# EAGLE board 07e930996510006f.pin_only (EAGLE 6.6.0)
REV: B

Size 45 x 85 mm. Coordinates in mm from the lower left corner, seen from the top.
Outline: 0,3 0,82 arc-90 3,85 42,85 arc-90 45,82 45,3 arc-90 42,0 3,0 arc-90 0,3
Copper layers (1*16): Top 0.035mm / dielectric 1.5mm / Bottom 0.035mm
Design rules "adafruit": minimum track width 8mil, minimum drill 15.5mil, track to track 8mil, track to pad 8mil, pad to pad 8mil, via to via 8mil, smd to smd 8mil, copper to edge 10mil, drill to drill 8mil, minimum pad ring 10mil, minimum via ring 8mil, stop-mask expansion 4mil, vias tented up to drill 20mil, thermal gap 10mil
tRestrict: area 31.5,16.2 to 31.9,16.3; area 4.2,24.6 to 4.5,24.6; area 4.2,31.8 to 4.6,31.9; area 4.2,16.8 to 4.6,16.9; area 4.2,16.2 to 4.6,16.2

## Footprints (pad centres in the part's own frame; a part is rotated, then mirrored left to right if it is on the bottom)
_0805 = smd 1.2 x 1.3: 1 -1.016,0; 2 1.016,0
PANASONIC_C = smd 2.6 x 1.4: + 2.05,0; - -2.05,0
POWERDI-5 = smd 1.39 x 1.4: A1 -0.92,-2.84; A2 0.92,-2.84 | smd 3.36 x 4.86: C 0,1.142
SOD-323 = smd 1.35 x 0.8: A 1.27,0; C -1.27,0
FIDUCIAL_1MM = smd 1 x 1: 1 0,0
SOIC8 = smd 0.5 x 2.2: 1 -1.905,-3.154; 2 -0.645,-3.154; 3 0.625,-3.154; 4 1.895,-3.154; 5 1.905,3.154; 6 0.635,3.154; 7 -0.635,3.154; 8 -1.905,3.154
AVRISP = drill 0.9 pad 1.626: 1 -1.27,2.54; 2 1.27,2.54; 3 -1.27,0; 4 1.27,0; 5 -1.27,-2.54; 6 1.27,-2.54
1X01-CLEANBIG = drill 1.016 pad 1.778: 1 0,0
INDUCTOR_6X6MM_SUMIDA_CDRH5D28 = smd 3 x 6.5: P$1 -2.075,0; P$2 2.075,0
INDUCTOR_5X5MM_TDK_VLC5045 = smd 2.54 x 5: P$1 -2.096,0; P$2 2.096,0
CHIPLED_0805 = smd 1.2 x 1.2: A 0,-1.05; C 0,1.05
EG1390 = smd 1 x 1.5: O1 -2.5,2.8; O2 -2.5,-2.8; P1 0,2.8; P2 0,-2.8; S1 2.5,2.8; S2 2.5,-2.8 | hole 1: 1.5,0; -1.5,0
DPAK = smd 1.6 x 2.997: 1 -2.261,-4.928; 3 2.21,-4.928 | smd 5.452 x 7: 4 0,1.853
_0805MP = smd 1.2 x 1.3: 1 -1.016,0; 2 1.016,0
2512 = smd 1.8 x 3.2: 1 -2.8,0; 2 2.8,0
SOLDERJUMPER_2WAY_OPEN_NOPASTE = smd 1.168 x 1.6: 1 -1.397,0; 2 0,0; 3 1.397,0
EVQ-Q2 = smd 3.2 x 1.2: A -3.4,-2; A' 3.4,-2; B -3.4,2; B' 3.4,2
SOT-23 = smd 0.787 x 0.889: 1 0.025,-1.016; 2 -0.94,1.016; 3 0.991,1.016
TESTPOINT_ROUND_1MM = smd 1 x 1: P$1 0,0
QFN32_5MM = smd 0.8 x 0.25: 1 -2.5,1.75; 2 -2.5,1.25; 3 -2.5,0.75; 4 -2.5,0.25; 5 -2.5,-0.25; 6 -2.5,-0.75; 7 -2.5,-1.25; 8 -2.5,-1.75; 17 2.5,-1.75; 18 2.5,-1.25; 19 2.5,-0.75; 20 2.5,-0.25; 21 2.5,0.25; 22 2.5,0.75; 23 2.5,1.25; 24 2.5,1.75 | smd 0.25 x 0.8: 9 -1.75,-2.5; 10 -1.25,-2.5; 11 -0.75,-2.5; 12 -0.25,-2.5; 13 0.25,-2.5; 14 0.75,-2.5; 15 1.25,-2.5; 16 1.75,-2.5; 25 1.75,2.5; 26 1.25,2.5; 27 0.75,2.5; 28 0.25,2.5; 29 -0.25,2.5; 30 -0.75,2.5; 31 -1.25,2.5; 32 -1.75,2.5 | smd 3.5 x 3.5: 33 0,0
QFN16_3MM = smd 0.8 x 0.28: 1 -1.5,0.75; 2 -1.5,0.25; 3 -1.5,-0.25; 4 -1.5,-0.75; 9 1.5,-0.75; 10 1.5,-0.25; 11 1.5,0.25; 12 1.5,0.75 | smd 0.28 x 0.8: 5 -0.75,-1.5; 6 -0.25,-1.5; 7 0.25,-1.5; 8 0.75,-1.5; 13 0.75,1.5; 14 0.25,1.5; 15 -0.25,1.5; 16 -0.75,1.5 | smd 1.5 x 1.5: THERMAL 0,0
MOUNTINGHOLE_3.0_PLATEDTHIN = drill 3 pad 3.6: P$1 0,0
DISPLAYPORT_0472720001 = smd 0.25 x 2.4: 1 5.5,10.28; 2 5,10.28; 3 4.5,10.28; 4 4,10.28; 5 3.5,10.28; 6 3,10.28; 7 2.5,10.28; 8 2,10.28; 9 1.5,10.28; 10 1,10.28; 11 0.5,10.28; 12 0,10.28; 13 -0.5,10.28; 14 -1,10.28; 15 -1.5,10.28; 16 -2,10.28; 17 -2.5,10.28; 18 -3,10.28; 19 -3.5,10.28; 20 -4,10.28 | drill 0.7 pad 1.4 long: P$2 8.25,0.9; P$3 -8.25,0.9; P$4 8.25,7.68; P$5 -8.25,7.68 | hole 1.4: 0,0
FPC_51PIN_502250-5191_EXT = smd 0.26 x 1.1: 1 7.5,-1.625; 3 6.9,-1.625; 5 6.3,-1.625; 7 5.7,-1.625; 9 5.1,-1.625; 11 4.5,-1.625; 13 3.9,-1.625; 15 3.3,-1.625; 17 2.7,-1.625; 19 2.1,-1.625; 21 1.5,-1.625; 23 0.9,-1.625; 25 0.3,-1.625; 27 -0.3,-1.625; 29 -0.9,-1.625; 31 -1.5,-1.625; 33 -2.1,-1.625; 35 -2.7,-1.625; 37 -3.3,-1.625; 39 -3.9,-1.625; 41 -4.5,-1.625; 43 -5.1,-1.625; 45 -5.7,-1.625; 47 -6.3,-1.625; 49 -6.9,-1.625; 51 -7.5,-1.625 | smd 0.3 x 0.95: 2 7.2,1.55; 4 6.6,1.55; 6 6,1.55; 8 5.4,1.55; 10 4.8,1.55; 12 4.2,1.55; 14 3.6,1.55; 16 3,1.55; 18 2.4,1.55; 20 1.8,1.55; 22 1.2,1.55; 24 0.6,1.55; 26 0,1.55; 28 -0.6,1.55; 30 -1.2,1.55; 32 -1.8,1.55; 34 -2.4,1.55; 36 -3,1.55; 38 -3.6,1.55; 40 -4.2,1.55; 42 -4.8,1.55; 44 -5.4,1.55; 46 -6,1.55; 48 -6.6,1.55; 50 -7.2,1.55
DCJACK_2MM_SMT = smd 2.4 x 2: GND 0,-5.5; GNDBREAK 6.2,-5.5; PWR 0,5.5; PWR2 6.2,5.5 | hole 1.6: 0,0 | hole 1.8: 4.5,0

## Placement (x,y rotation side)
C1  10uF  [_0805]  4,41 180 top
C2  4.7uF/50V  [_0805]  10.1,41.2 180 top
C3  4.7nF  [_0805]  21.5,33 180 top
C4  4.7uF/50V  [_0805]  18.1,52.7 270 top
C5  4.7uF/50V  [_0805]  19.9,52.7 270 top
C6  4.7uF/50V  [_0805]  21.7,52.7 270 top
C7  4.7uF/50V  [_0805]  23.5,52.7 270 top
C8  4.7uF/50V  [_0805]  25.3,52.7 270 top
C9  10uF/16V  [_0805]  40.9,50.5 270 top
C10  10uF/16V  [_0805]  43.4,50.5 270 top
C11  22nF  [_0805]  30.4,46.6 270 top
C12  10uF  [_0805]  41.66,45 90 top
C13  10uF  [_0805]  43.4,45 90 top
C14  0.1uF  [_0805]  38.1,44.96 90 top
C15  0.1uF  [_0805]  39.88,44.96 90 top
C16  47uF 25V  [PANASONIC_C]  16.64,64.39 0 top
D1  PDS560-13  [POWERDI-5]  21.5,57.5 270 top
D2  1N4148  [SOD-323]  34.92,69.34 270 top
FID1  FIDUCIAL""  [FIDUCIAL_1MM]  6.5,4.75 0 top
FID2  FIDUCIAL""  [FIDUCIAL_1MM]  38.43,83.34 0 top
FID3  FIDUCIAL""  [FIDUCIAL_1MM]  9.9,47.5 0 top
IC1  ATTINY85-20S  [SOIC8]  39.62,75.82 270 top
ISP1  AVRISP-6  [AVRISP]  40.01,69.47 90 top
JP1  [1X01-CLEANBIG]  21.84,67.06 0 top
L1  22uH  [INDUCTOR_6X6MM_SUMIDA_CDRH5D28]  5,46.5 90 top
L2  4.7uH (445-6526-1-ND)  [INDUCTOR_5X5MM_TDK_VLC5045]  38.3,38 0 top
LED1  green  [CHIPLED_0805]  6,10.5 270 top
ON/OFF  EG1390  [EG1390]  5.93,63.64 270 top
Q1  IRLR024NTRPBF  [DPAK]  11.4,56.6 270 top
R1  470  [_0805]  6,8.5 180 top
R2  100K  [_0805]  10.1,38.5 180 top
R3  100K  [_0805]  10.1,36.5 0 top
R4  20K  [_0805]  24.5,36 270 top
R5  27K  [_0805]  23.5,41 270 top
R6  20K  [_0805MP]  32.26,3.81 270 top
R7  20K  [_0805MP]  30.5,61.25 0 top
R8  47K  [_0805]  26.5,36 270 top
R9  20K  [_0805]  25.5,41 270 top
R10  47K  [_0805]  20.5,36 90 top
R11  15K  [_0805]  24.5,44 180 top
R12  7.5K  [_0805]  22.5,36 90 top
R13  0.058  [2512]  12.5,51 180 top
R14  20K  [_0805]  25.15,67.06 180 top
SJ1  [SOLDERJUMPER_2WAY_OPEN_NOPASTE]  39.04,33.81 180 top
SW1  SPST_TACT-EVQQ2  [EVQ-Q2]  13.97,73.66 90 top
SW2  SPST_TACT-EVQQ2  [EVQ-Q2]  5.33,73.66 270 top
SW3  SPST_TACT-EVQQ2  [EVQ-Q2]  27.94,73.66 90 top
T1  IRLML2246  [SOT-23]  30.5,64.5 270 top
T2  IRLML2246  [SOT-23]  36.58,3.81 90 top
TP1  GND  [TESTPOINT_ROUND_1MM]  25,63 90 top
TP2  VIN  [TESTPOINT_ROUND_1MM]  23,63 90 top
TP3  20V  [TESTPOINT_ROUND_1MM]  23,60.5 90 top
TP4  GND  [TESTPOINT_ROUND_1MM]  25,60.5 90 top
U1  LT3754  [QFN32_5MM]  17.1,42 270 top
U2  MCP16321T-330E/NG  [QFN16_3MM]  34.4,45.5 90 top
U$10  [SYMBOL_POSITIVE_CENTER-M]  28.53,57.15 270 top
U$11  MOUNTINGHOLE3.0THIN  [MOUNTINGHOLE_3.0_PLATEDTHIN]  42,3 0 top
U$32  MOUNTINGHOLE3.0THIN  [MOUNTINGHOLE_3.0_PLATEDTHIN]  42,82 0 top
U$33  MOUNTINGHOLE3.0THIN  [MOUNTINGHOLE_3.0_PLATEDTHIN]  3,82 0 top
U$34  MOUNTINGHOLE3.0THIN  [MOUNTINGHOLE_3.0_PLATEDTHIN]  3,3 0 top
U$39  [ADAFRUIT_TEXT_30MM]  28.96,1.91 90 top
X1  0472720001  [DISPLAYPORT_0472720001]  42,17 90 top
X2  502250-5191  [FPC_51PIN_502250-5191_EXT]  6,24 270 top
X3  2.1mm  [DCJACK_2MM_SMT]  43,59.5 180 top

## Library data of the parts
C1-C16 D1 D2 L1 L2 LED1 Q1 R1-R14 SJ1 TP1-TP4 U1 U2 U$10 U$39 X1-X3 = microbuilder
FID1-FID3 U$11 U$32-U$34 = microbuilder; BOM: EXCLUDE
IC1 = avr
ISP1 JP1 ON/OFF SW1-SW3 = adafruit
T1 T2 = zetex

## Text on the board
tPlace: PWM Backlight Control | Backlight | On/Off | UP | DOWN | On | Power | Off | 9-12VDC / 1000mA | LP097QX1 | Retina iPad / DisplayPort Driver / 9.7" 2048x1536 | POWER | DisplayPort

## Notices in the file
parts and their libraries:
microbuilder: This work is placed in the public domain, and may be freely used for commercial and non-commercial work with the following conditions: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
